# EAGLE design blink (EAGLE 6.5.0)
AUTHOR: Brad Campbell; REV: A; TITLE: Blink
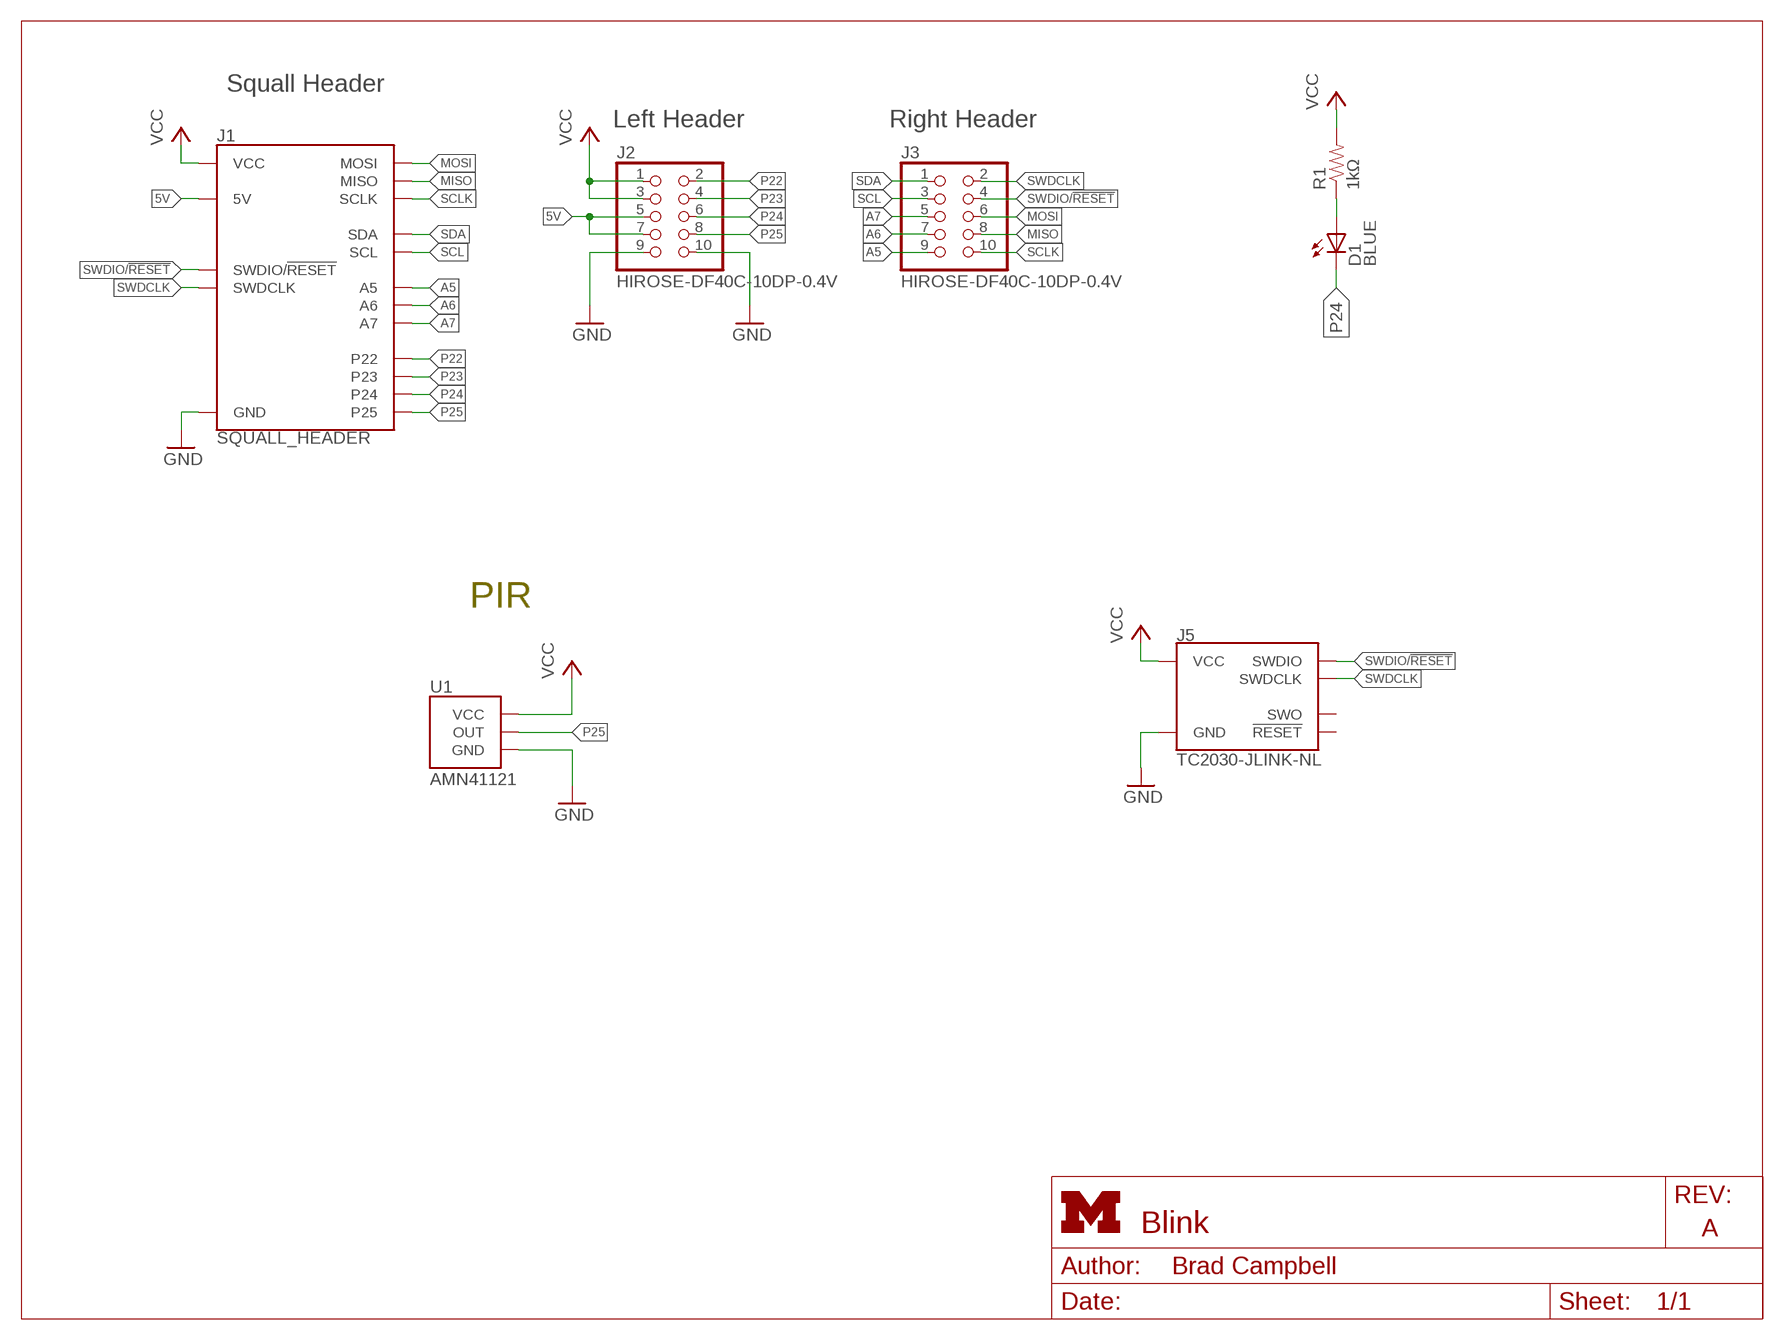
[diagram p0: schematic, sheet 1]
FRAME1 (LETTER_L): HEIGHT: 8.5in; WIDTH: 11in

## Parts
D1  BLUE  LED0603  [LED-0603]
J1  SQUALL_HEADER  [SQUALL_HEADER]
J2  HIROSE-DF40C-10DP-0.4V  [2X5/SMD/0.4MM]
J3  HIROSE-DF40C-10DP-0.4V  [2X5/SMD/0.4MM]
J5  TC2030-JLINK-NL  [TC2030-IDC-NL]
R1  1kΩ  RESISTOR0402_RES  [0402_RES]
U1  AMN41121  [AMN2]

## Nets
5V: J1.A5(5V) J1.A7(5V) J2.5 J2.7
A5: J1.B9(A5) J3.9
A6: J1.B7(A6) J3.7
A7: J1.B5(A7) J3.5
GND: J1.A9(GND) J1.A10(GND) J2.9 J2.10 J5.5(GND) U1.GND
MISO: J1.B8(MISO) J3.8
MOSI: J1.B6(MOSI) J3.6
N$2: D1.A R1.1
P22: J1.A2(P22) J2.2
P23: J1.A4(P23) J2.4
P24: D1.C J1.A6(P24) J2.6
P25: J1.A8(P25) J2.8 U1.OUT
SCL: J1.B3(SCL) J3.3
SCLK: J1.B10(SCLK) J3.10
SDA: J1.B1(SDA) J3.1
SWDCLK: J1.B2(SWDCLK) J3.2 J5.4(SWDCLK)
SWDIO/!RESET: J1.B4(SWDIO/!RESET) J3.4 J5.2(SWDIO)
VCC: J1.A1(VCC) J1.A3(VCC) J2.1 J2.3 J5.1(VCC) R1.2 U1.VCC
Unconnected: J5.3(!RESET) J5.6(SWO)

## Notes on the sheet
- Squall Header
- Left Header | Right Header
- PIR

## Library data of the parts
D1 = SparkFun-LED:LED: LEDs
J1 = squall:SQUALL_HEADER: Header for a sensor board on top of the Squall BLE tag board. Requires two DF40C-10DS-0.4V(51).; DIGIKEY: H11617CT-ND
J2 J3 = headers:HIROSE-DF40C-10DP-0.4V: DF40 Series Header - 0.4MM Pitch; DIGIKEY: H11616CT-ND; MOUSER: 798-DF40C10DP0.4V51; NEWARK: 68X2585
J5 = connector:TC2030-JLINK
R1 = passives:RESISTOR: Resistor
U1 = chips:AMN: Passive infrared human detection sensor with built-in amp.; DIGIKEY: 255-2651-ND

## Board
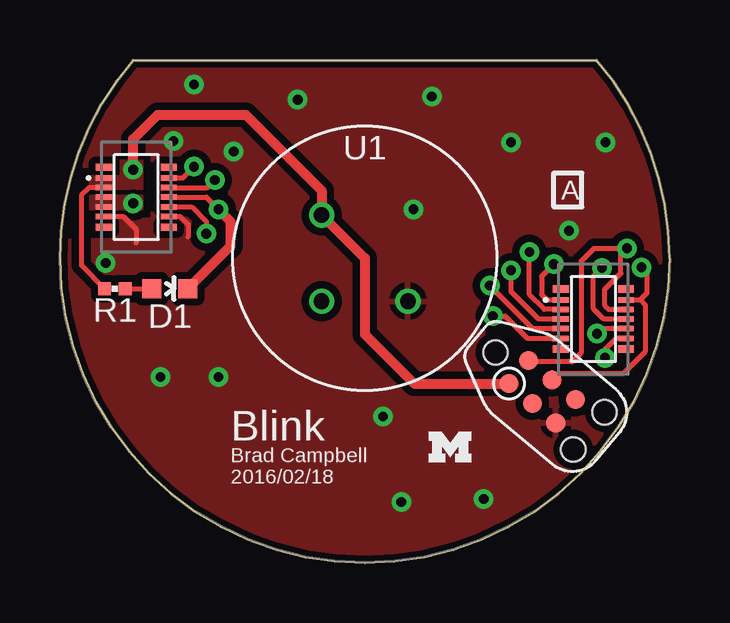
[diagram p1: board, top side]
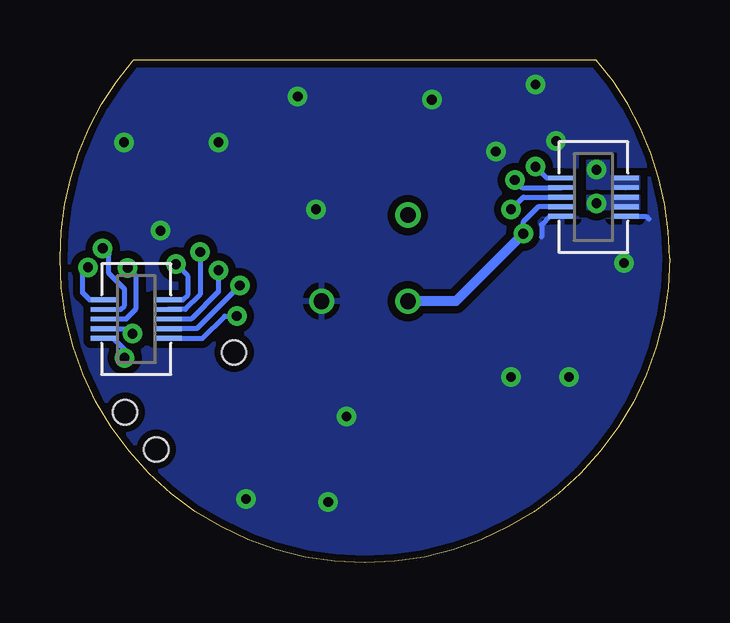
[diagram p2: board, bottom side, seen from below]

Size 25.4 x 20.95 mm. Coordinates in mm from the lower left corner, seen from the top.
Outline: 3.05,20.95 22.35,20.95 arc-41 25.4,12.7 arc-180 0,12.7 arc-41 3.05,20.95
Copper layers (1*16): Top 0.0178mm / dielectric 59mil / Bottom 0.0178mm
Design rules "sunstone-2lyr_v1.0.0.3 *": minimum track width 6mil, minimum drill 14mil, track to track 6mil, track to pad 6mil, pad to pad 6mil, via to via 6mil, smd to smd 6mil, copper to edge 10mil, drill to drill 16mil, minimum pad ring 8mil, minimum via ring 8mil, stop-mask expansion 3mil, vias tented up to drill 50mil, thermal gap 10mil

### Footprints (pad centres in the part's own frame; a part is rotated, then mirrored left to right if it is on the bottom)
LED-0603 = smd 0.8 x 0.8: A 0,-0.75; C 0,0.75
SQUALL_HEADER = smd 1.14 x 0.2 bottom: A1 -10.845,3.34; A2 -8.205,3.34; A3 -10.845,2.94; A4 -8.205,2.94; A5 -10.845,2.54; A6 -8.205,2.54; A7 -10.845,2.14; A8 -8.205,2.14; A9 -10.845,1.74; A10 -8.205,1.74; B1 8.205,-1.74; B2 10.845,-1.74; B3 8.205,-2.14; B4 10.845,-2.14; B5 8.205,-2.54; B6 10.845,-2.54; B7 8.205,-2.94; B8 10.845,-2.94; B9 8.205,-3.34; B10 10.845,-3.34
2X5/SMD/0.4MM = smd 0.66 x 0.23: 1 -1.355,0.8; 2 1.355,0.8; 3 -1.355,0.4; 4 1.355,0.4; 5 -1.355,0; 6 1.355,0; 7 -1.355,-0.4; 8 1.355,-0.4; 9 -1.355,-0.8; 10 1.355,-0.8 | smd 0.66 x 0.3: A -1.355,1.25; B 1.355,1.25; C -1.355,-1.25; D 1.355,-1.25
TC2030-IDC-NL = smd 0.787 x 0.787: 1 -1.27,-0.635; 2 -1.27,0.635; 3 0,-0.635; 4 0,0.635; 5 1.27,-0.635; 6 1.27,0.635 | hole 1.016: -2.54,0; 2.54,1.016; 2.54,-1.016
0402_RES = smd 0.536 x 0.546: 1 -0.433,0; 2 0.433,0
AMN2 = drill 0.65: GND 1.796,-1.796; OUT -1.796,-1.796; VCC -1.796,1.796

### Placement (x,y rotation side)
D1  4.57,11.43 270 top
J1  12.7,12.7 0 top
J2  3.17,15.24 0 top
J3  22.23,10.16 0 top
J5  20.09,7.14 320 top
R1  2.29,11.43 180 top
U1  12.7,12.7 0 top
U$1  [UMICH_SOLID_50MIL]  16.26,4.83 0 top

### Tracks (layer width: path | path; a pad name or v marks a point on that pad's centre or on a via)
5V  (via drill 0.41)
  other vias: 3.05,14.99
  pour Top (no thermals): 1.27,15.29 1.27,14.73 3.43,14.73 3.43,15.29
  pour Bottom (no thermals): 1.27,15.29 1.27,14.73 3.43,14.73 3.43,15.29
A5  (via drill 0.41)
  Top 0.203: v18.03,10.29 18.54,10.29 19.47,9.36 J3.9
  Bottom 0.203: J1.B9 19.47,9.36 18.54,10.29 v18.03,10.29
A6  (via drill 0.41)
  Top 0.203: J3.7 19.7,9.76 v17.91,11.56
  Bottom 0.203: J1.B7 19.7,9.76 v17.91,11.56
A7  (via drill 0.41)
  Top 0.203: J3.5 19.94,10.16 18.8,11.3 v18.8,12.19
  Bottom 0.203: v18.8,12.19 18.8,11.3 19.94,10.16 J1.B5
GND  (via drill 0.41)
  Top 0.203: J2.10 4.99,14.44 5.33,14.1 5.33,13.59 | J2.9 2.63,14.44 3.17,13.89 3.17,13.33
  Bottom 0.203: J1.A10 4.99,14.44 5.33,14.1 5.33,13.59 | J1.A9 0.98,14.44 0.86,14.33
  other vias: 4.72,17.58 1.9,12.5 9.91,19.3 15.49,19.43 18.8,17.53 22.73,17.53 17.65,2.67 14.22,2.54 6.6,7.75 4.19,7.75 14.73,14.73 5.59,19.94 7.24,17.14 21.21,13.84 13.46,6.1
  pour Top (isolate 0.305, rank 2): 25.4,12.7 arc-180 0,12.7 arc-41 3.05,20.95 22.35,20.95 arc-41
  pour Bottom (isolate 0.305, rank 2): 25.4,12.7 arc-180 0,12.7 arc-41 3.05,20.95 22.35,20.95 arc-41
MISO  (via drill 0.41)
  Top 0.203: J3.8 22.59,9.76 v22.38,9.55
  Bottom 0.203: J1.B8 22.59,9.76 v22.38,9.55
MOSI  (via drill 0.41)
  Top 0.203: J3.6 22.66,10.16 22.23,10.59 22.23,11.94 v22.58,12.29
  Bottom 0.203: J1.B6 22.66,10.16 22.23,10.59 22.23,11.94 v22.58,12.29
N$2
  Top 0.203: R1.1 D1.A
P22  (via drill 0.41)
  Top 0.203: J2.2 5.12,16.04 v5.59,16.51
  Bottom 0.203: v5.59,16.51 5.12,16.04 J1.A2
P23  (via drill 0.41)
  Top 0.203: J2.4 6.14,15.64 v6.45,15.95
  Bottom 0.203: v6.45,15.95 6.14,15.64 J1.A4
P24  (via drill 0.41)
  Top 0.203: J2.6 6.1,15.24 v6.6,14.73
  Top 0.406: D1.C 7.11,13.22 7.11,14.22 v6.6,14.73
  Bottom 0.203: v6.6,14.73 6.1,15.24 J1.A6
P25  (via drill 0.41)
  Top 0.203: J2.8 5.48,14.84 6.1,14.22 v6.1,13.72
  Bottom 0.203: J1.A8 5.48,14.84 6.1,14.22 v6.1,13.72
  Bottom 0.406: v6.1,13.72 8.91,10.9 U1.OUT
SCL  (via drill 0.41)
  Top 0.203: J3.3 20.17,10.56 19.56,11.18 v19.56,12.95
  Bottom 0.203: v19.56,12.95 19.56,11.18 20.17,10.56 J1.B3
SCLK  (via drill 0.41)
  Top 0.203: J3.10 23.18,9.36 22.71,8.89 v22.71,8.55
  Bottom 0.203: J1.B10 23.18,9.36 22.71,8.89 v22.71,8.55
SDA  (via drill 0.41)
  Top 0.203: v20.57,12.45 20.07,11.94 20.07,11.18 20.28,10.96 J3.1
  Bottom 0.203: J1.B1 20.28,10.96 20.07,11.18 20.07,11.94 v20.57,12.45
SWDCLK  (via drill 0.41)
  Top 0.203: J3.2 24.17,10.96 | 24.17,10.96 24.46,11.25 24.46,12.09 v24.23,12.32 | 24.17,10.96 24.38,10.74 24.38,8.8 23.47,7.89 20.76,7.89 J5.4
  Bottom 0.203: J1.B2 24.17,10.96 24.46,11.25 24.46,12.09 v24.23,12.32
SWDIO/!RESET  (via drill 0.41)
  Top 0.203: J3.4 22.86,10.57 22.71,10.72 22.71,11.4 23.37,12.06 23.37,12.85 v23.62,13.11 22.25,13.11 21.72,12.57 21.72,8.76 21.34,8.38 19.59,8.38 J5.2
  Bottom 0.203: J1.B4 22.87,10.56 22.71,10.72 22.71,11.4 23.37,12.06 23.37,12.85 v23.62,13.11
VCC  (via drill 0.41)
  Top 0.203: J2.3 1.21,15.64 0.89,15.32 0.89,12.39 R1.2
  Top 0.406: v3.05,16.38 3.05,17.65 4.06,18.67 7.75,18.67 10.9,15.51 U1.VCC 12.7,12.7 12.7,9.52 14.76,7.47 J5.1
  Bottom 0.203: J1.A3 J2.3
  pour Bottom (no thermals): 1.27,16.1 2.54,16.1 2.54,16.76 3.43,16.76 3.43,15.6 1.27,15.6
  pour Top (no thermals): 1.27,15.6 1.27,16.1 2.54,16.1 2.54,16.76 3.43,16.76 3.43,15.6

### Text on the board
tPlace: A | Blink | 2016/02/18 | Brad Campbell

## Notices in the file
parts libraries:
SparkFun-LED: Licensing: CC v3.0 Share-Alike You are welcome to use this library for commercial purposes.
